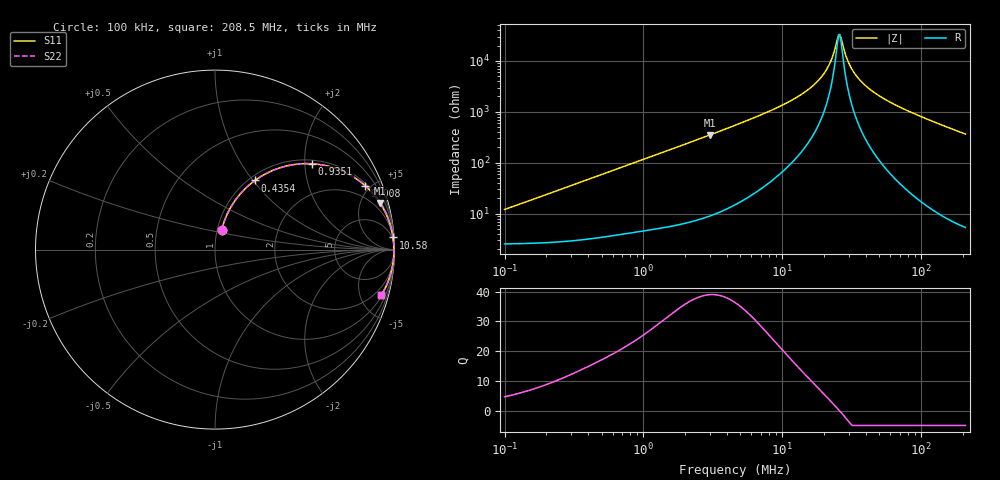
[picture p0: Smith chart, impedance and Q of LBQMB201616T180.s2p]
! LBQMB201616T180  S-PARAMETER MODEL  ( General Type )
! Model Generated by TAIYO YUDEN Corporation (http://www.ty-top.com)
! Version 1.0
! TAIYO YUDEN Control No. 191025NI43SB-FBB
! Copyright(c) 2019 TAIYO YUDEN CO.,LTD. All Rights Reserved.
! Product Description (link to TY-COMPAS)
! https://ds.yuden.co.jp/TYCOMPAS/or/detail?pn=LBQMB201616T180J&u=M
! Products Name : Inductors
! Characteristics :
!  Inductance : 18 uH , SRF(min) : 18 MHz , DC Resistance(max) : 3.25 Ohm , Rated Current : 150 mA
!  Case Size : 2.0 x 1.6 / 0.079 x 0.063 [mm/inch] , Thickness : 1.6 / 0.063 [mm/inch]
!  (Conditions: Temperature = 25 degC , DC Bias Current/Voltage = 0A / 0V)
! External Node Assignments :
!  1  o---GGG---o  2
! GND o---------o GND
! Frequency Range : 0.1MHz  -  208.503118MHz  [ 402 STEP ]
# MHz S RI R 50
! Freq[MHz].  S11 Real  S11 Imag  S21 Real  S21 Imag  S12 Real  S12 Imag  S22 Real  S22 Imag
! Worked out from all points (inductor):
!   401 points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, 100 kHz to 208.5 MHz, reference 50 ohm
!   read as one part in series: L = 18.9 uH near 103.9 kHz
!   highest Q = 39 at 2.999 MHz (marker M1), where L = 18.6 uH
!   self-resonance near 25.49 MHz
!   S11 on the Smith chart (normalised r, x): 100 kHz: 1.05, +0.24; 435.4 kHz: 1.07, +1.02; 935.1 kHz: 1.09, +2.18; 2.008 MHz: 1.13, +4.66; 10.58 MHz: 3, +29; 208.5 MHz: 1.11, -7.32
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0.1  0.0378 0.1112  0.9622 -0.1112  0.9622 -0.1112  0.0378 0.1112
0.206688  0.0786 0.2193  0.9214 -0.2193  0.9214 -0.2193  0.0786 0.2193
0.359709  0.1702 0.3413  0.8298 -0.3413  0.8298 -0.3413  0.1702 0.3413
0.435441  0.2228 0.3854  0.7772 -0.3854  0.7772 -0.3854  0.2228 0.3854
0.935062  0.5412 0.4783  0.4588 -0.4783  0.4588 -0.4783  0.5412 0.4783
1.293906  0.6874 0.4468  0.3126 -0.4468  0.3126 -0.4468  0.6874 0.4468
2.007944  0.838 0.3548  0.162 -0.3548  0.162 -0.3548  0.838 0.3548
2.999198  0.919 0.2603  0.081 -0.2603  0.081 -0.2603  0.919 0.2603
4.654297  0.9639 0.1731  0.0361 -0.1731  0.0361 -0.1731  0.9639 0.1731
10.58422  0.9918 0.0675  0.00815 -0.0675  0.00815 -0.0675  0.9918 0.0675
16.42508  0.9958 0.0313  0.00424 -0.0313  0.00424 -0.0313  0.9958 0.0313
18.77552  0.9964 0.0216  0.00364 -0.0216  0.00364 -0.0216  0.9964 0.0216
21.05614  0.9967 0.0137  0.00329 -0.0137  0.00329 -0.0137  0.9967 0.0137
22.72846  0.9969 0.00848  0.00313 -0.00848  0.00313 -0.00848  0.9969 0.00848
25.00684  0.997 0.00202  0.003 -0.00202  0.003 -0.00202  0.997 0.00202
25.98091  0.997 -0.000553  0.00297 0.000553  0.00297 0.000553  0.997 -0.000553
30.27169  0.997 -0.0109  0.003 0.0109  0.003 0.0109  0.997 -0.0109
34.60359  0.9968 -0.0202  0.0032 0.0202  0.0032 0.0202  0.9968 -0.0202
42.69694  0.996 -0.0356  0.00395 0.0356  0.00395 0.0356  0.996 -0.0356
59.08252  0.9935 -0.0628  0.00653 0.0628  0.00653 0.0628  0.9935 -0.0628
100.8781  0.982 -0.1228  0.018 0.1228  0.018 0.1228  0.982 -0.1228
208.5031  0.9273 -0.2524  0.0727 0.2524  0.0727 0.2524  0.9273 -0.2524
